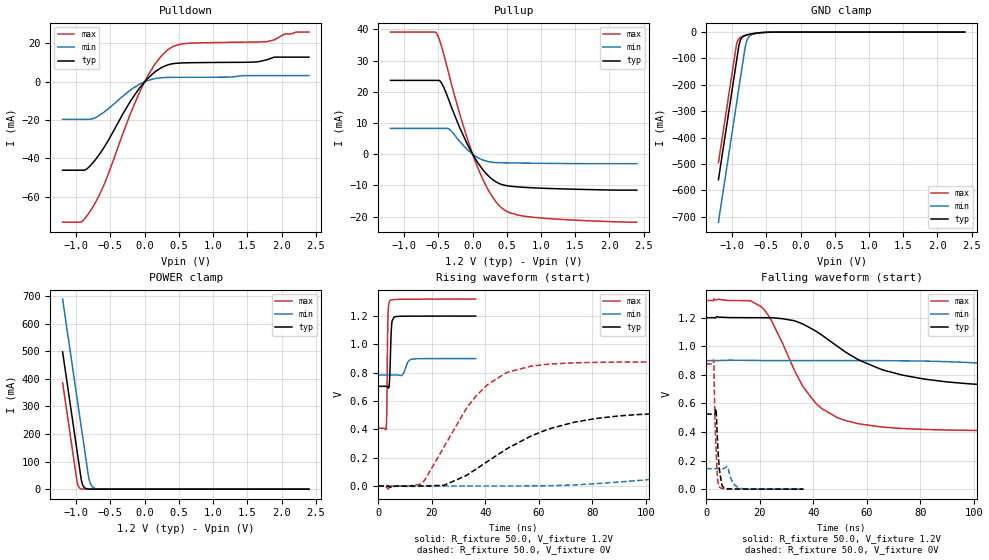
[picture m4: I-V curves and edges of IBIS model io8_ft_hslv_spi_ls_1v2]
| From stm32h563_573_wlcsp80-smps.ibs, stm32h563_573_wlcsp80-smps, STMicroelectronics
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[Model]   io8_ft_hslv_spi_ls_1v2
Model_type I/O
Polarity   Non-Inverting
Enable   Active-Low
| CAP_THRESHOLD on pad IOFT is "UDTCAPC" :
| Rising=20.0% of vddiom   Falling=80.0% of vddiom
| C_comp min and max val. don't necessarily correlate with the min and max pvt
| but are the smallest and greatest pad capacitance found.
| var   typ   min   max
C_comp   4.03040pF  3.93185pF  4.03600pF
|C_comp_pullup   2.46585pF  2.28015pF  2.18950pF
|C_comp_pulldown   1.56455pF  1.65170pF  1.84650pF
Vinl = 270.0mV
Vinh = 924.0mV
Vmeas = 600.0mV   | Reference voltage for timing measurements
Cref  = 50.0pF   | Timing specification test load capacitance value
Rref  = 100.0MOhm   | Timing specification test load resistance value
Vref  = 600.0mV   | Timing specification test load voltage
[Model Spec]
| TIME_THRESHOLD on pin ZIV11 is "CMOS" :
| Rising=40.0% of vdd   Falling=60.0% of vdd
Vinl 447.80000mV 344.80000mV 489.80000mV
Vinh 733.20000mV 535.20000mV 813.20000mV
| variable   typ   min   max
[Temperature Range] 25.0 125.0 -40.0
| variable   typ   min   max
[Voltage Range] 1.2V 900.0mV 1.32V
| variable   typ   min   max
[POWER Clamp Reference] 1.2V 900.0mV 1.32V
| variable   typ   min   max
[GND Clamp Reference] 0V 0V 0V
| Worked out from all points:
|   slope of the pulldown table from 0 to 0.18 V, typ, clamps not added: 30.6 ohm
|   slope of the pullup table from 0 to 0.18 V, typ, clamps not added: 31.3 ohm
|   GND clamp passes 1 mA (typ) near -0.52 V on its own axis
|   POWER clamp passes 1 mA (typ) near -0.84 V on its own axis
|   rising waveform, R_fixture 50.0, V_fixture 1.2V: 20-80 % time 527ps typ, 1.42ns min, 331ps max; typ from 0.704 V to 1.2 V
|   falling waveform, R_fixture 50.0, V_fixture 1.2V: 20-80 % time 30.9ns typ, 76.4ns min, 16.1ns max; typ from 1.2 V to 0.704 V
|   rising waveform, R_fixture 50.0, V_fixture 0V: 20-80 % time 31.7ns typ, 68.4ns min, 18.5ns max; typ from 0 V to 0.525 V
|   falling waveform, R_fixture 50.0, V_fixture 0V: 20-80 % time 1.13ns typ, 2.14ns min, 897ps max; typ from 0.525 V to 0 V
[POWER Clamp]
-1.2V     497.8mA    689.2mA    386.5mA
-990mV    140.8mA    332.2mA    29.53mA
-980mV    123.8mA    315.2mA    17.95mA
-960mV    89.81mA    281.2mA    6.634mA
-930mV    38.81mA    230.2mA    1.49mA
-900mV    12.07mA    179.2mA    334.8uA
-870mV    3.756mA    128.2mA    75.22uA
-820mV    536.4uA    44.98mA    6.246uA
-790mV    166.9uA    18.76mA    1.403uA
-750mV    35.18uA    5.846mA    191.9nA
-590mV    70.47nA    54.99uA    202.5pA
2.4V      0A         0A         0A
[GND Clamp]
-1.2V     -559.6mA   -720.6mA   -495.5mA
-940mV    -117.6mA   -278.6mA   -53.46mA
-930mV    -100.6mA   -261.6mA   -41.27mA
-900mV    -50.49mA   -210.6mA   -24.86mA
-880mV    -31.4mA    -176.6mA   -20.57mA
-850mV    -18.9mA    -125.6mA   -16.88mA
-810mV    -12.57mA   -58.3mA    -13.49mA
-780mV    -10.11mA   -29.57mA   -11.38mA
-740mV    -7.754mA   -14.31mA   -8.91mA
-640mV    -3.713mA   -4.821mA   -4.078mA
-390mV    -82.2uA    -288.6uA   -29.73uA
2.4V      3.859nA    727.3nA    172.3pA
| variable   typ   min   max
[Pullup Reference] 1.2V 900.0mV 1.32V
| variable   typ   min   max
[Pulldown Reference] 0V 0V 0V
[Pullup]
-1.2V     23.64mA    8.267mA    39.12mA
-550mV    23.64mA    8.267mA    39.12mA
-520mV    23.64mA    8.267mA    38.48mA
-450mV    22.64mA    8.267mA    34.23mA
-340mV    16.88mA    8.001mA    25.06mA
-200mV    9.064mA    4.383mA    13.74mA
40mV      -1.481mA   -615.3uA   -2.353mA
250mV     -7.344mA   -2.474mA   -12.27mA
450mV     -9.868mA   -2.757mA   -17.63mA
670mV     -10.5mA    -2.844mA   -19.55mA
920mV     -10.81mA   -2.91mA    -20.29mA
2.4V      -11.52mA   -3.043mA   -21.79mA
[Pulldown]
-1.2V     -46.17mA   -19.62mA   -73.27mA
-930mV    -46.17mA   -19.62mA   -73.17mA
-770mV    -42.8mA    -19.4mA    -66.04mA
-570mV    -32.88mA   -15.18mA   -51.58mA
-200mV    -9.658mA   -4.083mA   -15.89mA
-80mV     -3.488mA   -1.363mA   -5.887mA
140mV     4.817mA    1.545mA    8.585mA
340mV     8.782mA    2.25mA     16.66mA
540mV     9.805mA    2.305mA    19.74mA
1.79V     11.49mA    3.197mA    20.93mA
2.05V     12.83mA    3.197mA    24.95mA
2.4V      12.83mA    3.197mA    25.89mA
[Ramp]
dV/dt_r 315.11049mV/31.36969ns 85.96137mV/68.28432ns 525.76999mV/18.19374ns
dV/dt_f 297.79722mV/30.80665ns 69.60167mV/75.94465ns 547.13923mV/15.97046ns
R_load = 50.0
| Removed startup time: 0s 0s 0s  .
| Removed end time: 36.4ns.
[Rising Waveform]
R_fixture   = 50.0
V_fixture   = 1.2V
V_fixture_min = 900.0mV
V_fixture_max = 1.32V
0s        703.7mV    783.5mV    408.1mV
3ns       703.8mV    783.5mV    410.2mV
3.2ns     704mV      783.5mV    524.9mV
3.5ns     701.5mV    783.5mV    1.043V
3.65ns    697.2mV    783.5mV    1.192V
4.35ns    792.3mV    783.5mV    1.308V
5ns       1.132V     783.5mV    1.314V
5.95ns    1.193V     783.5mV    1.316V
12.65ns   1.199V     895.6mV    1.319V
36.4ns    1.2V       899.8mV    1.32V
| Removed startup time: 0s 0s 0s  .
| Removed end time: 399.4ns.
[Falling Waveform]
R_fixture   = 50.0
V_fixture   = 1.2V
V_fixture_min = 900.0mV
V_fixture_max = 1.32V
0s        1.2V       900mV      1.32V
20.2ns    1.2V       900.2mV    1.282V
24.45ns   1.2V       899.9mV    1.179V
36.25ns   1.155V     900mV      715.5mV
40.75ns   1.109V     900mV      605.5mV
48.9ns    1.001V     900mV      501.1mV
65.2ns    839.6mV    899.5mV    436mV
89.65ns   751.1mV    892.5mV    414mV
130.5ns   713.1mV    849.2mV    408.6mV
399.4ns   703.7mV    784mV      408.1mV
| Removed startup time: 0s 0s 0s  .
| Removed end time: 399.4ns.
[Rising Waveform]
R_fixture   = 50.0
V_fixture   = 0V
V_fixture_min = 0V
V_fixture_max = 0V
0s        166.4nV    851nV      114.4nV
16.1ns    -141.3uV   -35.43uV   18.07mV
24.6ns    5.594mV    -52.63uV   276.7mV
32.6ns    71.39mV    2.157uV    537.5mV
40.8ns    173.4mV    205.2uV    715.4mV
62ns      390.6mV    1.697mV    857.3mV
81.5ns    477.2mV    16.83mV    873.1mV
114.1ns   517mV      65.22mV    876mV
195.7ns   524.9mV    132.6mV    876.2mV
399.4ns   525.2mV    143.3mV    876.3mV
| Removed startup time: 0s 0s 0s  .
| Removed end time: 36.4ns.
[Falling Waveform]
R_fixture   = 50.0
V_fixture   = 0V
V_fixture_min = 0V
V_fixture_max = 0V
0s        525.3mV    143.5mV    876.3mV
2.8ns     525.4mV    143.5mV    904.4mV
3.25ns    527.4mV    143.5mV    526.5mV
3.9ns     492.8mV    143.5mV    198.2mV
4.35ns    302mV      143.6mV    61.79mV
4.95ns    145.1mV    143.5mV    16.55mV
5.95ns    24.86mV    143.4mV    4.573mV
7.45ns    4.242mV    154.4mV    2.791mV
12.65ns   781uV      7.173mV    1.115mV
36.4ns    329.1uV    65.88uV    133.7uV
